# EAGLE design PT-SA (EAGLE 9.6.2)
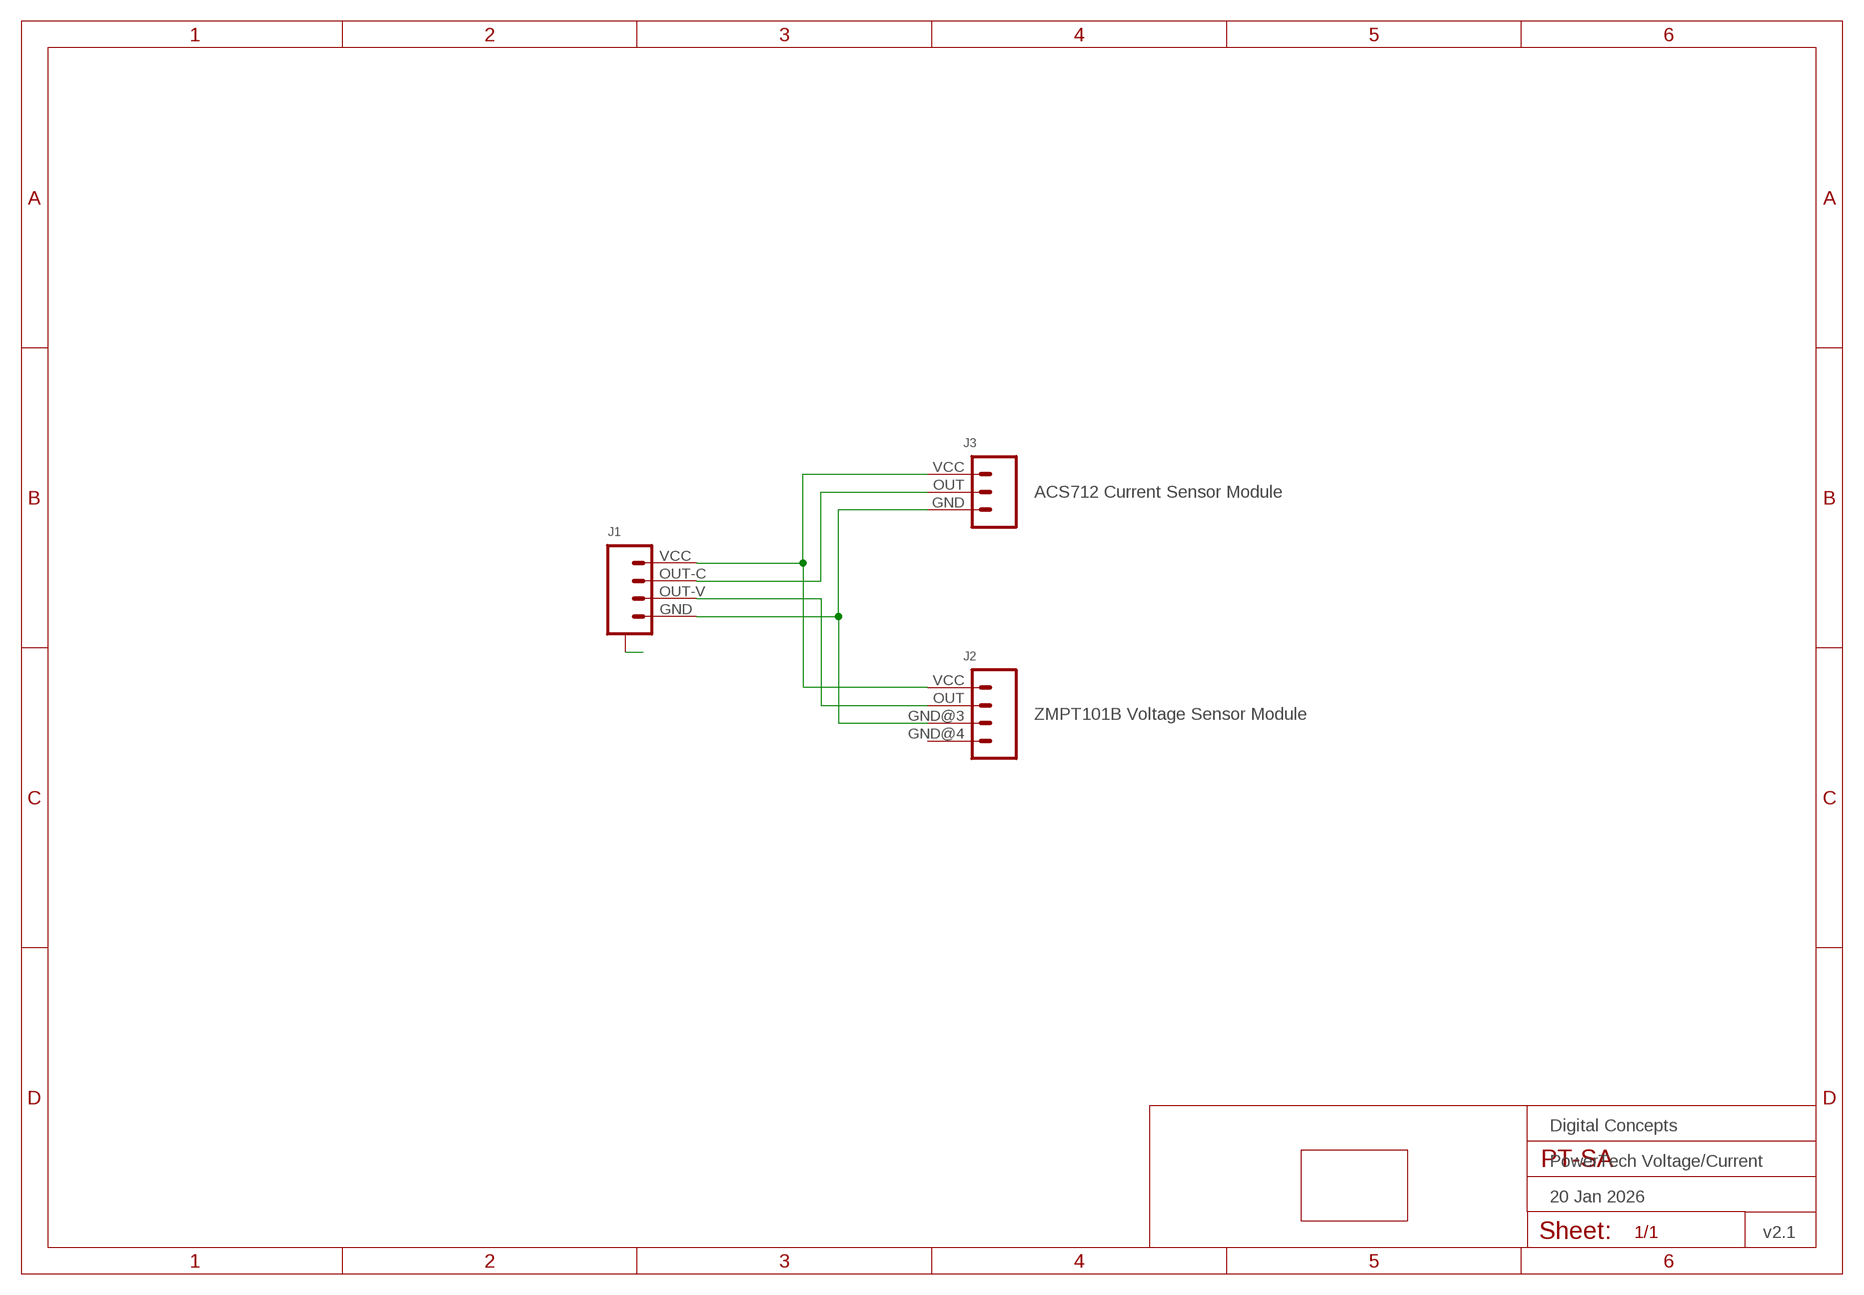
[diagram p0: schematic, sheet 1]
FRAME2 (FRAME-A4L-LOC): DATE: 20 Jan 2026; OWNER: Digital Concepts; TITLE: PowerTech Voltage/Current; VERSION: v2.1

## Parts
J1  JST-SH1.0-4-SMD-HORIZONTAL-POWERTECH  [JST-SH1.0-4-HORIZONTAL-POWERTECH]
J2  ZMPT101B Voltage Sensor Module  HEADER-1X4-ZMPT101B  [CONN_04-ZMPT101B]
J3  ACS712 Current Sensor Module  HEADER-1X3-ACS712  [CONN_03-ACS712]
PCB1  POWERTECH-SOCKET  [PCB-POWERTECH]

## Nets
A: J1.A@1(A) J1.A@4(A)
N$1: J1.VCC J2.VCC J3.VCC
N$2: J1.OUT-C J3.OUT
N$3: J1.OUT-V J2.OUT
N$4: J1.GND J2.GND@3 J3.GND
Unconnected: J2.GND@4

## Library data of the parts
J1 = digitalconcepts:JST-SH1.0-4-SMD-HORIZONTAL-POWERTECH: JST SH1.0 4P SMD horizontal connector - PowerTech
J2 = digitalconcepts:HEADER-1X4-ZMPT101B: Single Row 4-Pin Header
J3 = digitalconcepts:HEADER-1X3-ACS712: ACS712 Module Single Row 3-Pin Header
PCB1 = digitalconcepts:POWERTECH-SOCKET: PowerTech Socket Outlet Adaptor PCB

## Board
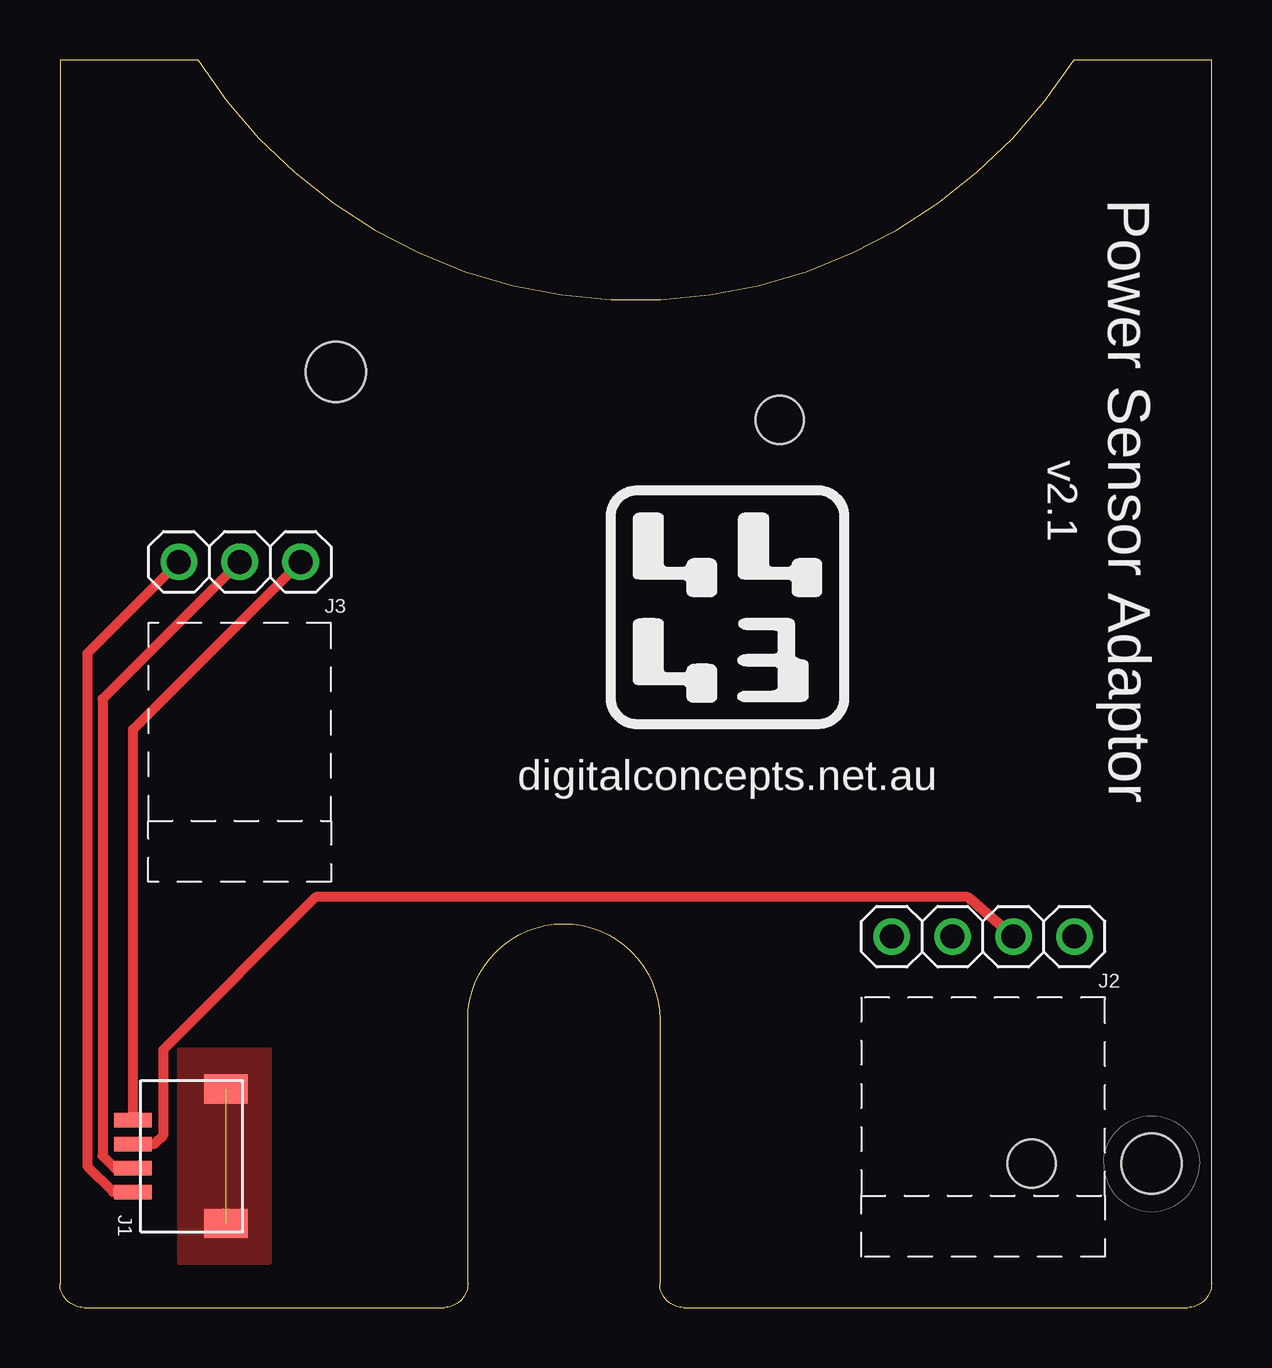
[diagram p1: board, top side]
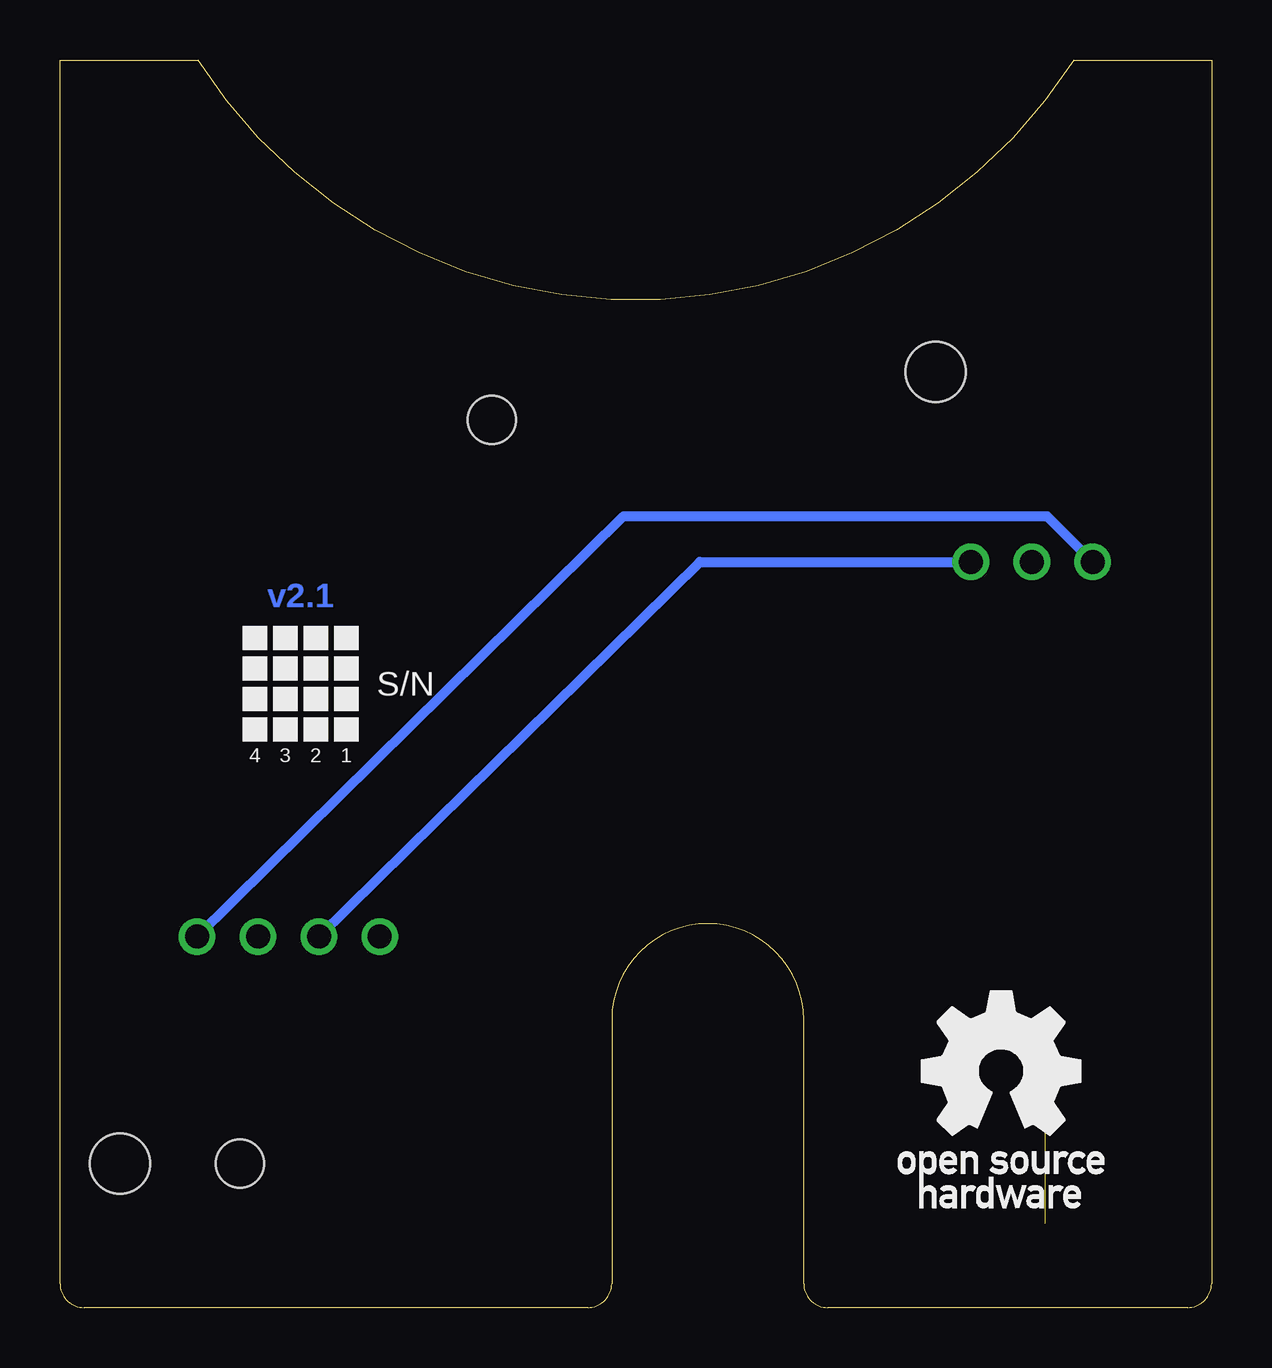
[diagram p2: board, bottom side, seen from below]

Size 48 x 52 mm. Coordinates in mm from the lower left corner, seen from the top.
Copper layers (1*16): Top 0.035mm / dielectric 1.5mm / Bottom 0.035mm
Design rules "default *": minimum track width 6mil, minimum drill 0.35mm, track to track 6mil, track to pad 6mil, pad to pad 6mil, via to via 6mil, smd to smd 6mil, copper to edge 6mil, drill to drill 6mil, minimum pad ring 10mil, minimum via ring 8mil, stop-mask expansion 4mil, vias tented up to drill 0mil, thermal gap 10mil

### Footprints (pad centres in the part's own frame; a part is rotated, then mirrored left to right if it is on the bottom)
JST-SH1.0-4-HORIZONTAL-POWERTECH = smd 1.2 x 1.8: A@1 -2.8,-1.335; A@4 2.8,-1.335 | smd 0.6 x 1.55: GND 1.5,2.54; OUT-C -0.5,2.54; OUT-V 0.5,2.54; VCC -1.5,2.54
CONN_04-ZMPT101B = drill 1 pad 1.524: GND@3 5.08,0; GND@4 7.62,0; OUT 2.54,0; VCC 0,0
CONN_03-ACS712 = drill 1 pad 1.524: GND 5.08,0; OUT 2.54,0; VCC 0,0
PCB-POWERTECH = hole 2.5: -20,-21.5; 13,12.5 | hole 2: -20,-16.5; 11,-6

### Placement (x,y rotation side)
J1  5.59,6.31 90 top
J2  42.29,15.46 180 top
J3  4.95,31.08 0 top
PCB1  24,26 90 top

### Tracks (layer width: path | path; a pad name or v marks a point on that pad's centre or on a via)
A  (1 unrouted)
  pour Top (no thermals): 4.95,10.76 8.76,10.76 8.76,1.87 4.95,1.87
N$1
  Top 0.406: J3.VCC 1.14,27.27 1.14,5.89 2.21,4.81 J1.VCC
  Bottom 0.406: J2.VCC 24.51,32.98 6.86,32.98 J3.VCC
N$2
  Top 0.406: J3.OUT 1.78,25.36 1.78,6.31 2.28,5.81 J1.OUT-C
N$3
  Top 0.406: J1.OUT-V 3.93,6.81 4.32,7.2 4.32,10.76 10.67,17.11 37.84,17.11 J2.OUT
N$4
  Top 0.406: J1.GND 3.05,24.09 J3.GND
  Bottom 0.406: J2.GND@3 21.33,31.08 J3.GND

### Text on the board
Bottom: v2.1
tPlace: v2.1 | Power Sensor Adaptor | digitalconcepts.net.au
bPlace: S/N | 1 | 2 | 3 | 4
